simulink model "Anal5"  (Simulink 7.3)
settings: Solver=ode45  StartTime=0.0  StopTime=10.0  RelTol=1e-3
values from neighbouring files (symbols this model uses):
  d2r = 1/r2d    (= 0.0174532925199)    [run.m]
  Kl3 = INFO.KFI(:,1:7)    [run.m]
  Kp3 = INFO.KFI(:,1:5)    [run.m]
  Thr = [470000, 470000, 470000, 0.245e7, 0.245e7]'    [run.m]
undefined symbols (not defined in the file or in its folder): Ap, Bp, Cp, Cyb, Cza, Dp, Mass, Qbar, Sref, TVC

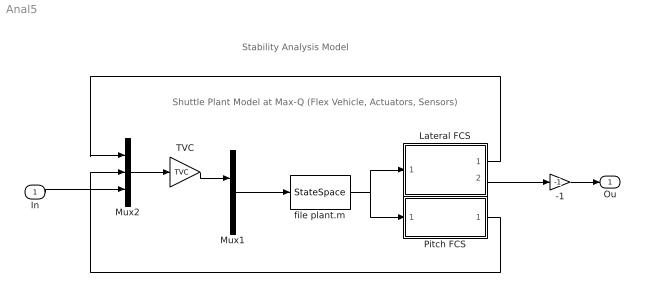
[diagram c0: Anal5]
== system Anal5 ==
  note: Shuttle Plant Model at Max-Q (Flex Vehicle, Actuators, Sensors)
  note: Stability Analysis Model
  In : Inport  OutDataType=sfix(16)  OutScaling=2^0
  -1 : Gain  Gain=-1  ParameterDataType=sfix(16)  ParameterScaling=2^0  OutDataType=sfix(16)  OutScaling=2^0
  Lateral FCS : Subsystem
  Mux1 : Mux  Inputs=[10,1]
  Mux2 : Mux  Inputs=3
  Pitch FCS : Subsystem
  TVC : Gain  Gain=TVC  Multiplication=Matrix(K*u)  ParameterDataType=sfix(16)  ParameterScaling=2^0  OutDataType=sfix(16)  OutScaling=2^0
  file plant.m : StateSpace  A=Ap  B=Bp  C=Cp  D=Dp
  Ou : Outport  OutDataType=sfix(16)  OutScaling=2^0
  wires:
  Mux1/1 -> file plant.m/1
  file plant.m/1 -> Lateral FCS/1(ym), Pitch FCS/1(ym)
  Mux2/1 -> TVC/1
  TVC/1 -> Mux1/1
  -1/1 -> Ou/1
  Lateral FCS/2(dR) -> -1/1
  In/1 -> Mux2/3
  Pitch FCS/1(dQ) -> Mux2/2
  Lateral FCS/1(dP) -> Mux2/1

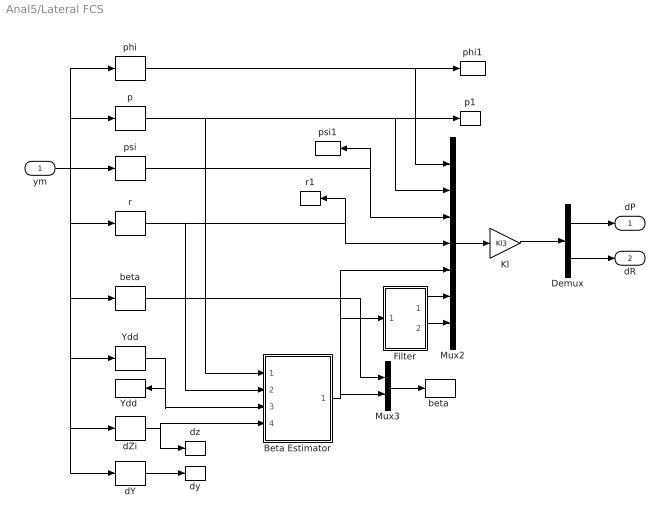
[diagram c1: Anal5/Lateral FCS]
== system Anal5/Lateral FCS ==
  ym : Inport
  Beta Estimator : Subsystem
  Demux : Demux  Outputs=2
  Filter : Subsystem
  Kl : Gain  Gain=Kl3  Multiplication=Matrix(K*u)  ParameterDataType=sfix(16)  ParameterScaling=2^0  OutDataType=sfix(16)  OutScaling=2^0
  Mux2 : Mux  Inputs=7
  Mux3 : Mux  Inputs=2
  Ydd : Selector  InputPortWidth=30  IndexOptions=Index vector (dialog)  Indices=[7]  OutputSizes=1
  "Ydd " : ToWorkspace  VariableName=Ydd  SampleTime=-1  SaveFormat=Array
  beta : Selector  InputPortWidth=30  IndexOptions=Index vector (dialog)  Indices=[10]  OutputSizes=1
  "beta " : ToWorkspace  VariableName=beta  SampleTime=-1  SaveFormat=Array
  dY : Selector  InputPortWidth=30  IndexOptions=Index vector (dialog)  Indices=[21:25]  OutputSizes=1
  dZi : Selector  InputPortWidth=30  IndexOptions=Index vector (dialog)  Indices=[26:30]  OutputSizes=1
  dy : ToWorkspace  VariableName=dy  SampleTime=-1  SaveFormat=Array
  dz : ToWorkspace  VariableName=dz  SampleTime=-1  SaveFormat=Array
  p : Selector  InputPortWidth=30  IndexOptions=Index vector (dialog)  Indices=[4]  OutputSizes=1
  p1 : ToWorkspace  VariableName=p  SampleTime=-1  SaveFormat=Array
  phi : Selector  InputPortWidth=30  IndexOptions=Index vector (dialog)  Indices=[1]  OutputSizes=1
  phi1 : ToWorkspace  VariableName=phi  SampleTime=-1  SaveFormat=Array
  psi : Selector  InputPortWidth=30  IndexOptions=Index vector (dialog)  Indices=[3]  OutputSizes=1
  psi1 : ToWorkspace  VariableName=psi  SampleTime=-1  SaveFormat=Array
  r : Selector  InputPortWidth=30  IndexOptions=Index vector (dialog)  Indices=[6]  OutputSizes=1
  r1 : ToWorkspace  VariableName=r  SampleTime=-1  SaveFormat=Array
  dP : Outport
  dR : Outport  Port=2
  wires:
  Demux/1 -> dP/1
  Demux/2 -> dR/1
  Kl/1 -> Demux/1
  dY/1 -> dy/1
  Mux3/1 -> "beta "/1
  Beta Estimator/1(bethat) -> Mux3/2, Mux2/5, Filter/1(bet)
  dZi/1 -> dz/1, Beta Estimator/4(dz)
  Ydd/1 -> "Ydd "/1, Beta Estimator/3(Ydd)
  ym/1 -> r/1, beta/1, Ydd/1, dZi/1, dY/1, psi/1, phi/1, p/1
  r/1 -> r1/1, Mux2/4, Beta Estimator/2(r)
  psi/1 -> psi1/1, Mux2/3
  p/1 -> p1/1, Mux2/2, Beta Estimator/1(p)
  phi/1 -> phi1/1, Mux2/1
  Filter/2(x2) -> Mux2/7
  Filter/1(x1) -> Mux2/6
  Mux2/1 -> Kl/1
  beta/1 -> Mux3/1

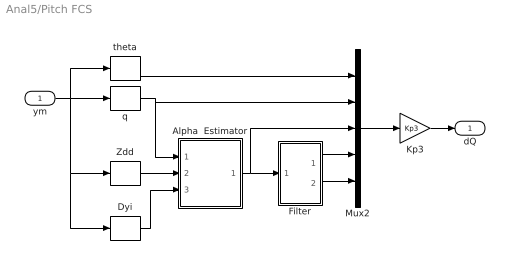
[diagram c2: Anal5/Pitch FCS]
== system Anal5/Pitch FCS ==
  ym : Inport
  Alpha  Estimator : Subsystem
  Dyi : Selector  InputPortWidth=30  IndexOptions=Index vector (dialog)  Indices=[21:25]  OutputSizes=1
  Filter : Subsystem
  Kp3 : Gain  Gain=Kp3  Multiplication=Matrix(K*u)  ParameterDataType=sfix(16)  ParameterScaling=2^0  OutDataType=sfix(16)  OutScaling=2^0
  Mux2 : Mux  Inputs=5
  Zdd : Selector  InputPortWidth=30  IndexOptions=Index vector (dialog)  Indices=[8]  OutputSizes=1
  q : Selector  InputPortWidth=30  IndexOptions=Index vector (dialog)  Indices=[5]  OutputSizes=1
  theta : Selector  InputPortWidth=30  IndexOptions=Index vector (dialog)  Indices=[2]  OutputSizes=1
  dQ : Outport
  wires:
  Mux2/1 -> Kp3/1
  Filter/1(x1) -> Mux2/4
  Filter/2(x2) -> Mux2/5
  theta/1 -> Mux2/1
  q/1 -> Mux2/2, Alpha  Estimator/1(q)
  ym/1 -> Zdd/1, Dyi/1, q/1, theta/1
  Alpha  Estimator/1(alphat) -> Filter/1(alfa), Mux2/3
  Zdd/1 -> Alpha  Estimator/2(Zdd)
  Dyi/1 -> Alpha  Estimator/3(delta)
  Kp3/1 -> dQ/1

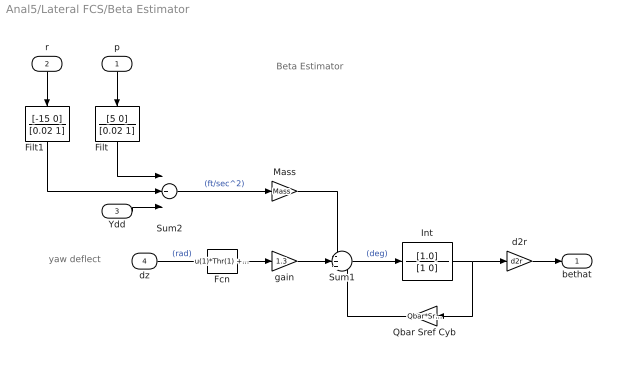
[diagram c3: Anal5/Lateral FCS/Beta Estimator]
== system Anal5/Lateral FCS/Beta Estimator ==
  note: yaw deflect
  note: Beta Estimator
  p : Inport
  r : Inport  Port=2
  Ydd : Inport  Port=3
  dz : Inport  Port=4  OutDataType=sfix(16)  OutScaling=2^0
  Fcn : Fcn  Expr=u(1)*Thr(1) +u(2)*Thr(2) +u(3)*Thr(3) +u(4)*Thr(4) +u(5)*Thr(5)
  Filt : TransferFcn  Numerator=[5 0]  Denominator=[0.02 1]
  Filt1 : TransferFcn  Numerator=[-15 0]  Denominator=[0.02 1]
  Int : TransferFcn  Numerator=[1.0]  Denominator=[1 0]
  Mass : Gain  Gain=Mass  ParameterDataType=sfix(16)  ParameterScaling=2^0  OutDataType=sfix(16)  OutScaling=2^0
  Qbar Sref Cyb : Gain  Gain=Qbar*Sref*Cyb  ParameterDataType=sfix(16)  ParameterScaling=2^0  OutDataType=sfix(16)  OutScaling=2^0
  Sum1 : Sum  Inputs=-++  OutDataType=sfix(16)  OutScaling=2^0
  Sum2 : Sum  Inputs=+++  OutDataType=sfix(16)  OutScaling=2^0
  d2r : Gain  Gain=d2r  ParameterDataType=sfix(16)  ParameterScaling=2^0  OutDataType=sfix(16)  OutScaling=2^0
  gain : Gain  Gain=1.3  ParameterDataType=sfix(16)  ParameterScaling=2^0  OutDataType=sfix(16)  OutScaling=2^0
  bethat : Outport  OutDataType=sfix(16)  OutScaling=2^0
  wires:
  Filt/1 -> Sum2/1
  p/1 -> Filt/1
  r/1 -> Filt1/1
  Ydd/1 -> Sum2/3
  gain/1 -> Sum1/2
  Fcn/1 -> gain/1
  Int/1 -> Qbar Sref Cyb/1, d2r/1
  d2r/1 -> bethat/1
  Mass/1 -> Sum1/1
  Sum2/1 -> Mass/1  "(ft/sec^2)"
  dz/1 -> Fcn/1  "(rad)"
  Qbar Sref Cyb/1 -> Sum1/3
  Sum1/1 -> Int/1  "(deg)"
  Filt1/1 -> Sum2/2

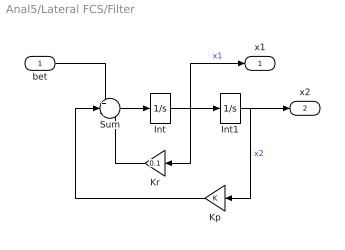
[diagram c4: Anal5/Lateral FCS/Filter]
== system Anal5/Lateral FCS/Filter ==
  bet : Inport  OutDataType=sfix(16)  OutScaling=2^0
  Int : Integrator
  Int1 : Integrator
  Kp : Gain  ParameterDataType=sfix(16)  ParameterScaling=2^0  OutDataType=sfix(16)  OutScaling=2^0
  Kr : Gain  Gain=0.1  ParameterDataType=sfix(16)  ParameterScaling=2^0  OutDataType=sfix(16)  OutScaling=2^0
  Sum : Sum  Inputs=+--  OutDataType=sfix(16)  OutScaling=2^0
  x1 : Outport  OutDataType=sfix(16)  OutScaling=2^0
  x2 : Outport  Port=2  OutDataType=sfix(16)  OutScaling=2^0
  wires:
  bet/1 -> Sum/1
  Kp/1 -> Sum/2
  Kr/1 -> Sum/3
  Int1/1 -> x2/1, Kp/1  "x2"
  Sum/1 -> Int/1
  Int/1 -> x1/1, Kr/1, Int1/1  "x1"

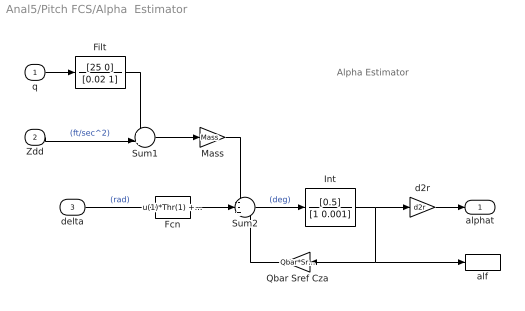
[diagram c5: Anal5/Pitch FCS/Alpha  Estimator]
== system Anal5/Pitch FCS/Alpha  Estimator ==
  note: Alpha Estimator
  q : Inport  OutDataType=sfix(16)  OutScaling=2^0
  Zdd : Inport  Port=2  OutDataType=sfix(16)  OutScaling=2^0
  delta : Inport  Port=3  OutDataType=sfix(16)  OutScaling=2^0
  Fcn : Fcn  Expr=u(1)*Thr(1) +u(2)*Thr(2) +u(3)*Thr(3) +u(4)*Thr(4) +u(5)*Thr(5)
  Filt : TransferFcn  Numerator=[25 0]  Denominator=[0.02 1]
  Int : TransferFcn  Numerator=[0.5]  Denominator=[1 0.001]
  Mass : Gain  Gain=Mass  ParameterDataType=sfix(16)  ParameterScaling=2^0  OutDataType=sfix(16)  OutScaling=2^0
  Qbar Sref Cza : Gain  Gain=Qbar*Sref*Cza  ParameterDataType=sfix(16)  ParameterScaling=2^0  OutDataType=sfix(16)  OutScaling=2^0
  Sum1 : Sum  Inputs=++|  OutDataType=sfix(16)  OutScaling=2^0
  Sum2 : Sum  Inputs=--+  OutDataType=sfix(16)  OutScaling=2^0
  alf : ToWorkspace  VariableName=alphat  SampleTime=-1  SaveFormat=Array
  d2r : Gain  Gain=d2r  ParameterDataType=sfix(16)  ParameterScaling=2^0  OutDataType=sfix(16)  OutScaling=2^0
  alphat : Outport  OutDataType=sfix(16)  OutScaling=2^0
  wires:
  Int/1 -> alf/1, Qbar Sref Cza/1, d2r/1
  d2r/1 -> alphat/1
  Mass/1 -> Sum2/1
  delta/1 -> Fcn/1  "(rad)"
  Qbar Sref Cza/1 -> Sum2/3
  Sum2/1 -> Int/1  "(deg)"
  q/1 -> Filt/1
  Zdd/1 -> Sum1/2  "(ft/sec^2)"
  Sum1/1 -> Mass/1
  Filt/1 -> Sum1/1
  Fcn/1 -> Sum2/2

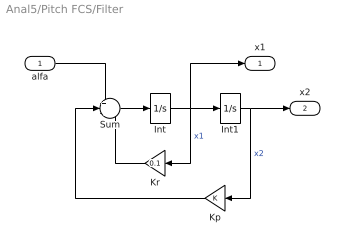
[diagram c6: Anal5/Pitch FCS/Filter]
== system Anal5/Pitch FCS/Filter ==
  alfa : Inport  OutDataType=sfix(16)  OutScaling=2^0
  Int : Integrator
  Int1 : Integrator
  Kp : Gain  ParameterDataType=sfix(16)  ParameterScaling=2^0  OutDataType=sfix(16)  OutScaling=2^0
  Kr : Gain  Gain=0.1  ParameterDataType=sfix(16)  ParameterScaling=2^0  OutDataType=sfix(16)  OutScaling=2^0
  Sum : Sum  Inputs=+--  OutDataType=sfix(16)  OutScaling=2^0
  x1 : Outport  OutDataType=sfix(16)  OutScaling=2^0
  x2 : Outport  Port=2  OutDataType=sfix(16)  OutScaling=2^0
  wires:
  Int/1 -> Int1/1, Kr/1, x1/1  "x1"
  Sum/1 -> Int/1
  Int1/1 -> Kp/1, x2/1  "x2"
  Kr/1 -> Sum/3
  Kp/1 -> Sum/2
  alfa/1 -> Sum/1
